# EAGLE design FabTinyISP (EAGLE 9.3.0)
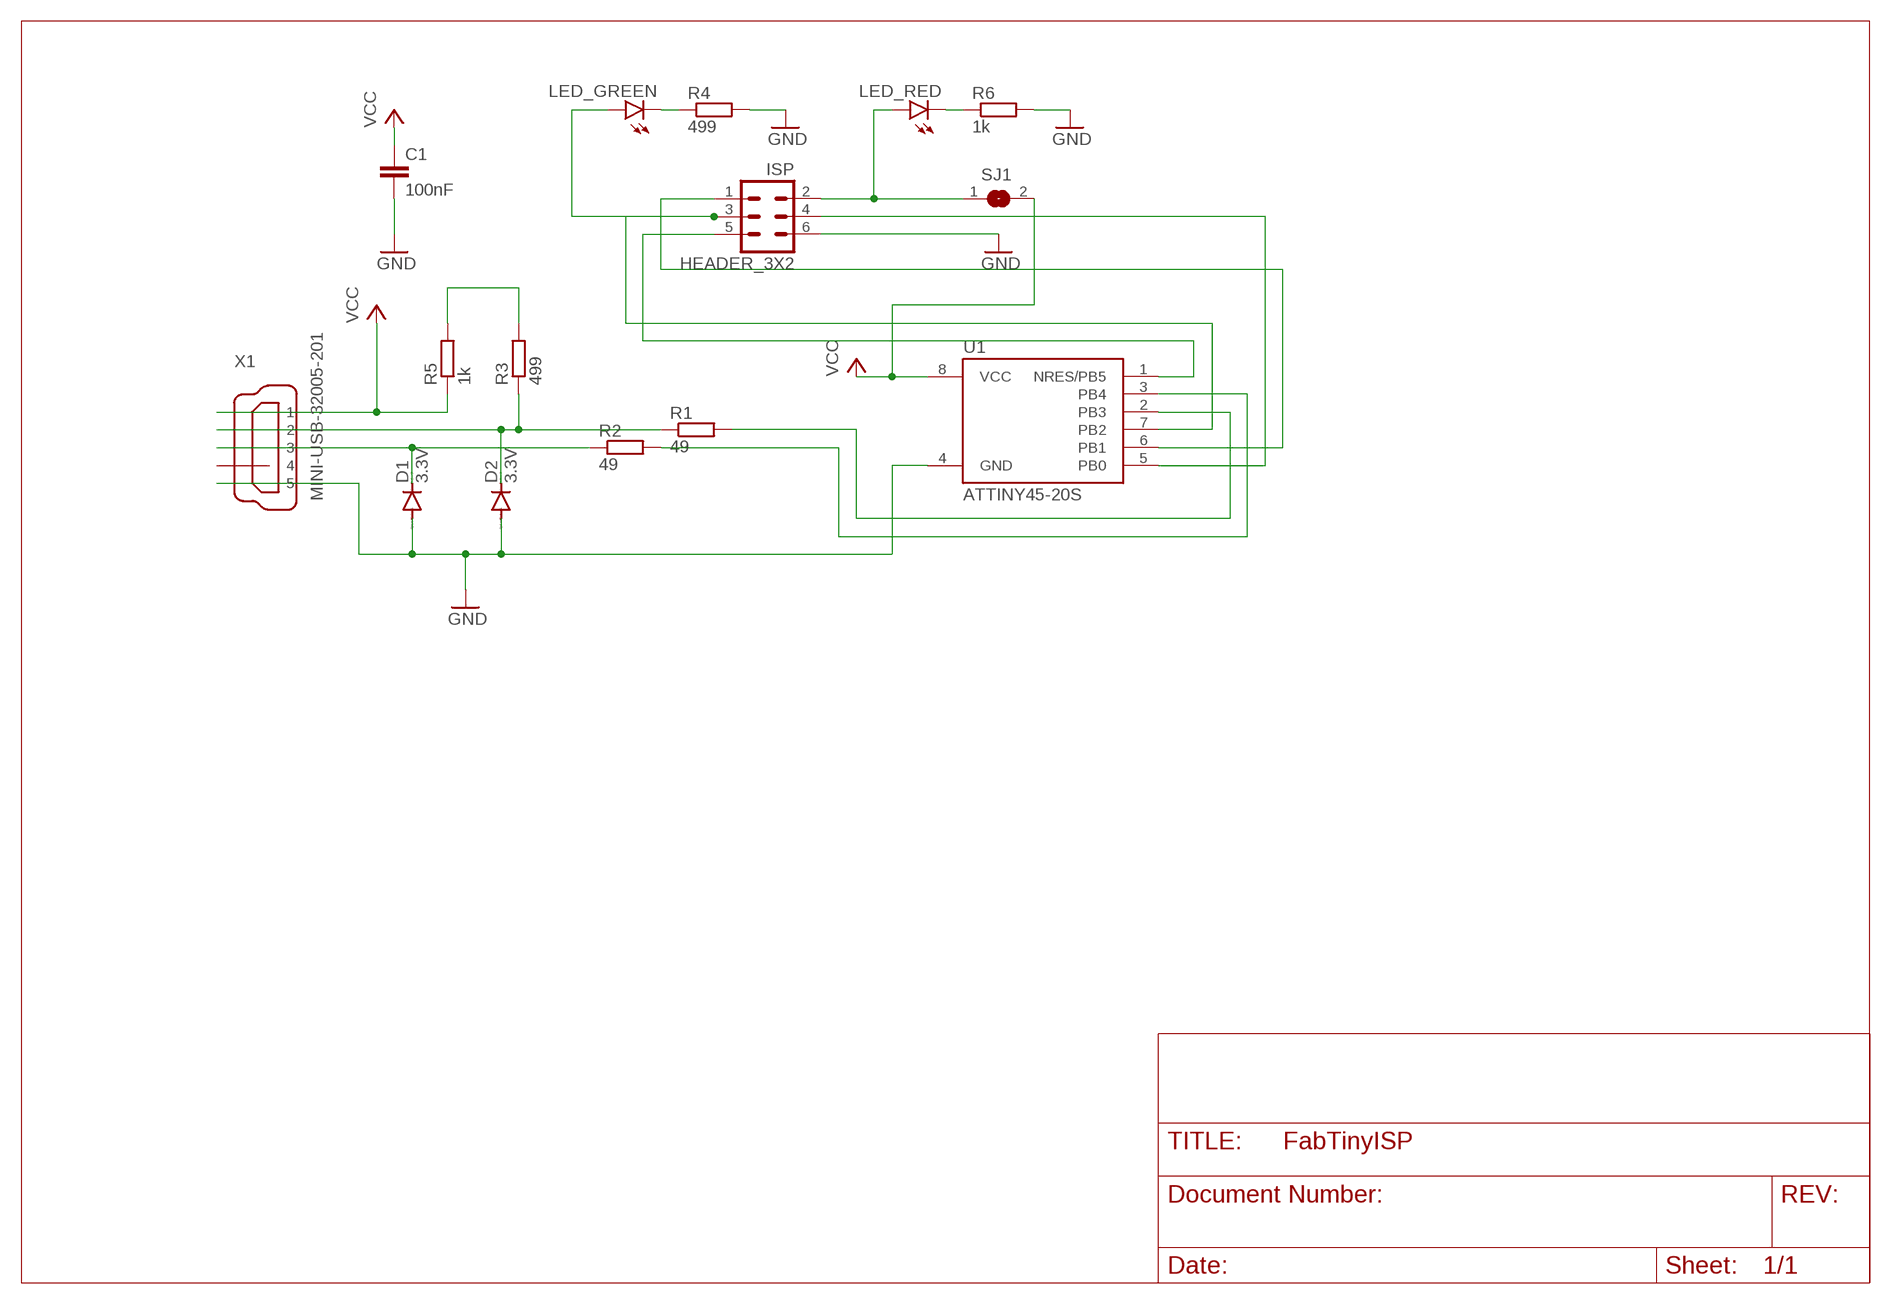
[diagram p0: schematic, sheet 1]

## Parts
C1  100nF  C-EUC0603  [C0603]
D1  3.3V  DIODE-MINIMELF  [MINIMELF]
D2  3.3V  DIODE-MINIMELF  [MINIMELF]
HEADER_3X2  ISP  MA03-2  [MA03-2]
LED_GREEN  LEDCHIP-LED0603  [CHIP-LED0603]
LED_RED  LEDCHIP-LED0603  [CHIP-LED0603]
R1  49  R-EU_R1206  [R1206]
R2  49  R-EU_R1206  [R1206]
R3  499  R-EU_R1206  [R1206]
R4  499  R-EU_R1206  [R1206]
R5  1k  R-EU_R1206  [R1206]
R6  1k  R-EU_R1206  [R1206]
SJ1  SJ  [SJ]
U1  ATTINY45-20S  [SOIC8_EIAJ_208MIL]
X1  MINI-USB-32005-201  [32005-201]

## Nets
GND: C1.2 D1.A D2.A HEADER_3X2.6 R4.2 R6.2 U1.4(GND) X1.5
N$1: D2.C R1.1 R3.1 X1.2
N$2: D1.C R2.1 X1.3
N$3: LED_GREEN.C R4.1
N$5: HEADER_3X2.2 LED_RED.A SJ1.1
N$6: R3.2 R5.2
N$7: HEADER_3X2.5 U1.1(NRES/PB5)
N$8: HEADER_3X2.3 LED_GREEN.A U1.7(PB2)
N$10: LED_RED.C R6.1
N$12: R1.2 U1.2(PB3)
N$13: R2.2 U1.3(PB4)
N$14: HEADER_3X2.4 U1.5(PB0)
N$15: HEADER_3X2.1 U1.6(PB1)
VCC: C1.1 R5.1 SJ1.2 U1.8(VCC) X1.1
Unconnected: X1.4

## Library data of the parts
C1 = rcl:C-EU: CAPACITOR, European symbol; SPICEPREFIX: C
D1 D2 = diode:DIODE-: DIODE
HEADER_3X2 = con-lstb:MA03-2: PIN HEADER; OC_FARNELL: unknown; OC_NEWARK: unknown
LED_GREEN LED_RED = led:LED: LED
R1-R6 = rcl:R-EU_: RESISTOR, European symbol; SPICEPREFIX: R
SJ1 = jumper:SJ: SMD solder JUMPER
U1 = _hhn_attiny25_45_85:ATTINY45*: ATMEL ATtiny 45 Packages: P = PDIP 08 30mil S = SOIC 08 EIAJ 208mil X = TSSOP 08 4.4mm Technologies Note: for complete ordering code (temp. range, finish, tape&reel etc.) see www.atmel.com &bull; Supply Voltage: V = (1.8&hellip;5.5)V | [blank] = (2.7&hellip;5.5)V &bull; Speed: 10 = 10 MHz | 20 = 20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
X1 = con-cypressindustries:MINI-USB-: MINI USB-B Conector Source: www.cypressindustries.com; OC_FARNELL: unknown; OC_NEWARK: unknown

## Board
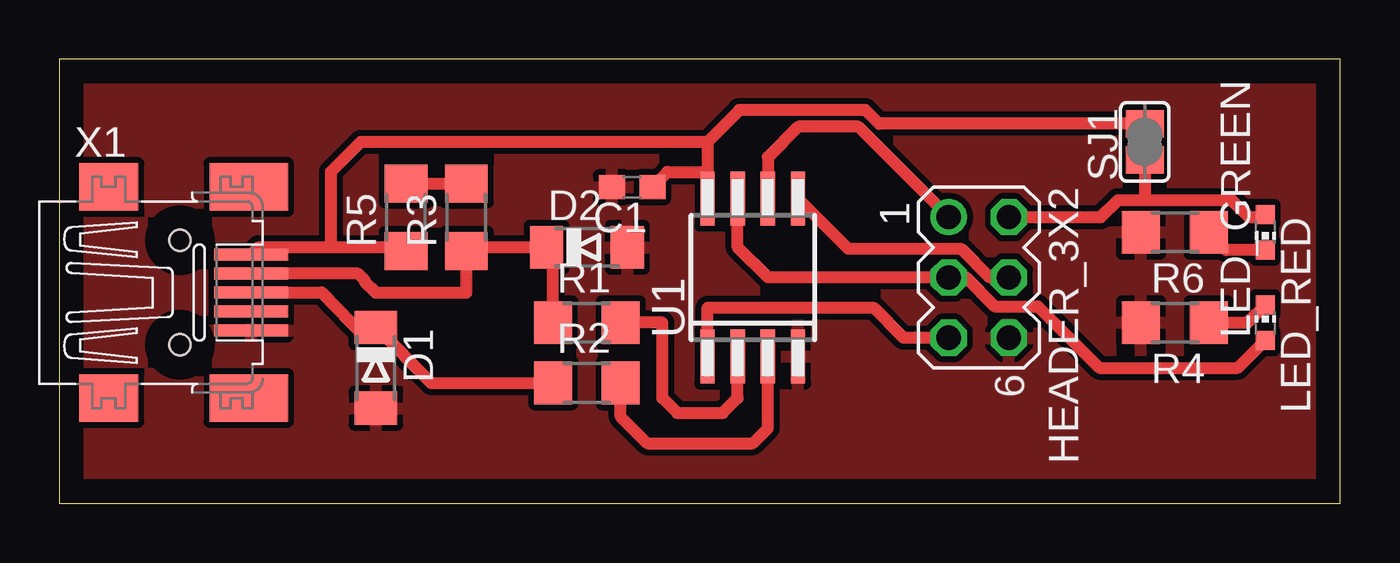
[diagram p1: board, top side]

Size 53.95 x 18.72 mm. Coordinates in mm from the lower left corner, seen from the top.
Outline: 0,0 53.95,0 53.95,18.72 0,18.72 0,0
Copper layers (1*16): Top 0.035mm / dielectric 1.5mm / Bottom 0.035mm
Design rules "default *": minimum track width 0.2mm, minimum drill 0.35mm, track to track 0.25mm, track to pad 0.25mm, pad to pad 0.25mm, via to via 0.25mm, smd to smd 0.25mm, copper to edge 40mil, drill to drill 6mil, minimum pad ring 10mil, minimum via ring 8mil, stop-mask expansion 4mil, vias tented up to drill 0mil, thermal gap 10mil

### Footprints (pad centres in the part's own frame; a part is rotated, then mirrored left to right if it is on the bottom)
C0603 = smd 1.1 x 1: 1 -0.85,0; 2 0.85,0
MINIMELF = smd 1.4 x 1.8: A 1.7,0; C -1.7,0
MA03-2 = drill 1.016: 1 -2.54,-1.27 | drill 1.016 octagon: 2 -2.54,1.27; 3 0,-1.27; 4 0,1.27; 5 2.54,-1.27; 6 2.54,1.27
CHIP-LED0603 = smd 0.8 x 0.8: A 0,-0.75; C 0,0.75
R1206 = smd 1.6 x 1.803: 1 -1.422,0; 2 1.422,0
SJ = smd 1.168 x 1.6: 1 -0.762,0; 2 0.762,0
SOIC8_EIAJ_208MIL = smd 0.6 x 2.286: 1 -1.905,-3.33; 2 -0.635,-3.33; 3 0.635,-3.33; 4 1.905,-3.33; 5 1.905,3.33; 6 0.635,3.33; 7 -0.635,3.33; 8 -1.905,3.33
32005-201 = smd 3.1 x 0.5: 1 3,1.6; 2 3,0.8; 3 3,0; 4 3,-0.8; 5 3,-1.6 | smd 2.5 x 2: M1 -3,-4.45; M2 -3,4.45 | smd 3.3 x 2: M3 2.9,4.45; M4 2.9,-4.45 | hole 0.9: 0,2.2; 0,-2.2

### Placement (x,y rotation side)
C1  24.13,13.34 180 top
D1  13.34,5.71 270 top
D2  22.22,10.79 0 top
HEADER_3X2  38.73,9.52 270 top
LED_GREEN  50.8,7.62 0 top
LED_RED  50.8,11.43 180 top
R1  22.22,7.62 0 top
R2  22.22,5.08 0 top
R3  17.14,12.07 90 top
R4  46.99,7.62 180 top
R5  14.61,12.07 90 top
R6  46.99,11.43 180 top
SJ1  45.72,15.24 90 top
U1  29.21,9.52 0 top
X1  5.08,8.89 0 top

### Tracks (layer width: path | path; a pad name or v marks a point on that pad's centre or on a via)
GND
  pour Top: -15.24,38.1 151.13,38.1 151.13,-77.47 -15.24,-77.47
N$1
  Top 0.508: R3.1 17.16,10.64 | 17.16,10.64 17.77,10.62 | 17.77,10.62 17.8,10.62 | R1.1 20.8,10.52 D2.C 17.95,10.79 17.77,10.62 | X1.2 12.58,9.69 12.88,9.39 12.88,9.34 13.34,8.89 17.14,8.89 17.14,10.62 17.16,10.64
N$2
  Top 0.508: 20.32,5.08 R2.1 15.67,5.08 D1.C 12.9,6.98 11.05,8.9 9.41,8.9 X1.3
N$3
  Top 0.508: R4.1 50.05,7.62 LED_GREEN.C
N$5
  Top 0.508: LED_RED.A 50.69,12.07 50.12,12.07 49.4,12.79 45.72,12.79 | HEADER_3X2.2 43.86,12.07 44.58,12.79 45.72,12.79 | SJ1.1 45.72,12.79
N$6
  Top 0.508: R5.2 R3.2
N$7
  Top 0.508: HEADER_3X2.5 35.56,6.98 34.29,8.26 27.31,8.26 U1.1
N$8
  Top 0.508: U1.7 28.57,10.79 29.85,9.52 HEADER_3X2.3 38.18,9.52 39.4,8.31 41.22,8.31 43.81,5.71 49.64,5.71 LED_GREEN.A
N$10
  Top 0.508: LED_RED.C 49.16,10.68 R6.1
N$12
  Top 0.508: R1.2 25.4,7.62 25.4,4.45 26.04,3.81 27.94,3.81 28.57,4.45 U1.2
N$13
  Top 0.508: U1.3 29.85,3.18 29.21,2.54 24.77,2.54 23.65,3.66 R2.2
N$14
  Top 0.508: HEADER_3X2.4 39.19,9.52 37.97,10.74 33.23,10.74 U1.5
N$15
  Top 0.508: HEADER_3X2.1 33.66,15.87 31.11,15.87 29.85,14.6 U1.6
VCC
  Top 0.508: 45.85,15.87 SJ1.2 34.53,16 33.95,16.58 28.65,16.58 27.31,15.24 | 27.31,15.24 27.31,13.97 | 27.31,13.97 U1.8 | X1.1 8.39,10.79 11.43,10.79 | 11.43,10.79 13.82,10.79 13.97,10.64 R5.1 | 27.31,15.24 12.7,15.24 11.43,13.97 11.43,10.79 | C1.1 25.61,13.97 27.31,13.97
